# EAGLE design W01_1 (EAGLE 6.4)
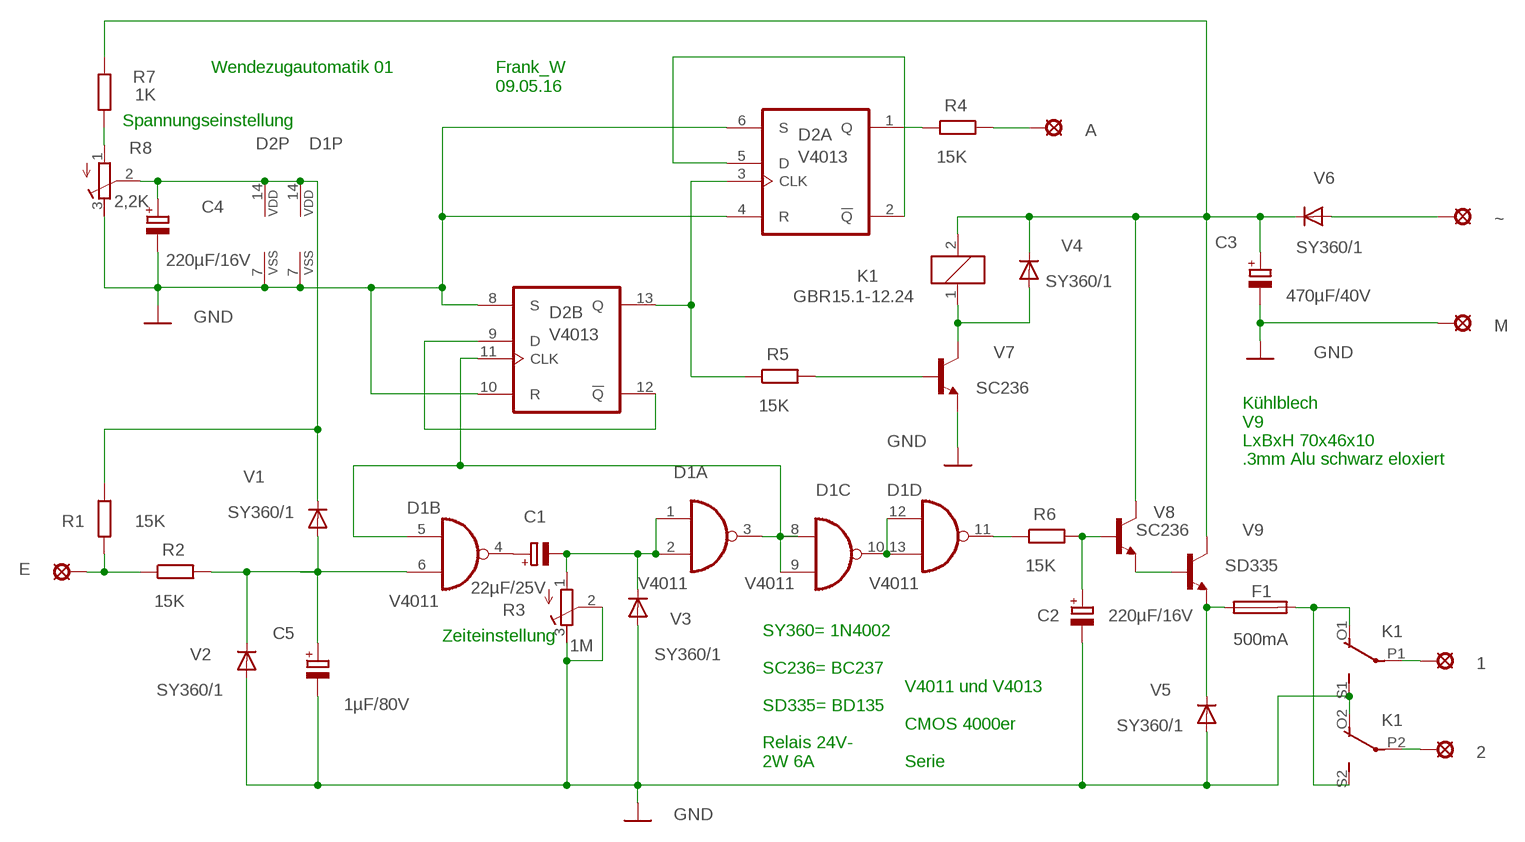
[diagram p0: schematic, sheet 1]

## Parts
1  LSP10  [LSP10]
2  LSP10  [LSP10]
A  LSP10  [LSP10]
C1  22µF/25V  CPOL-EUE5-5  [E5-5]
C2  220µF/16V  CPOL-EUE22-9AXIAL  [E22-9]
C3  470µF/40V  CPOL-EUE22-9AXIAL  [E22-9]
C4  220µF/16V  CPOL-EUE22-9AXIAL  [E22-9]
C5  1µF/80V  CPOL-EUE5-5  [E5-5]
D1  V4011  4011N  [DIL14]
D2  V4013  4013N  [DIL14]
E  LSP10  [LSP10]
F1  500mA  GSH15  [GSH15]
K1  GBR15.1-12.24  4052  [F4052]
M  LSP10  [LSP10]
R1  15K  R-EU_0207/12  [0207/12]
R2  15K  R-EU_0207/12  [0207/12]
R3  1M  R-TRIMM3296P  [RTRIM3296P]
R4  15K  R-EU_0207/12  [0207/12]
R5  15K  R-EU_0207/12  [0207/12]
R6  15K  R-EU_0207/12  [0207/12]
R7  1K  R-EU_0207/12  [0207/12]
R8  2,2K  R-TRIMM3296P  [RTRIM3296P]
V1  SY360/1  1N4004  [DO41-10]
V2  SY360/1  1N4004  [DO41-10]
V3  SY360/1  1N4004  [DO41-10]
V4  SY360/1  1N4004  [DO41-10]
V5  SY360/1  1N4004  [DO41-10]
V6  SY360/1  1N4004  [DO41-10]
V7  SC236  BC237  [TO92]
V8  SC236  BC237  [TO92]
V9  SD335  BD139  [TO126]
~  LSP10  [LSP10]

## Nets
GND: C2.- C3.- C4.- C5.- D1.7(P:VSS) D2.4(A:R) D2.6(A:S) D2.7(P:VSS) D2.8(B:S) D2.10(B:R) K1.O2(3:O) K1.S1(2:S) M.MP R3.2(S) R3.3(E) R8.3(E) V2.A V3.A V5.A V7.1(E)
N$1: E.MP R1.2 R2.1
N$2: C5.+ D1.6(B:I1) R2.2 V1.A V2.C
N$4: D2.9(B:D) D2.12(B:!Q)
N$6: D1.11(D:O) R6.1
N$7: C2.+ R6.2 V8.2(B)
N$8: R7.2 R8.1(A)
N$9: V6.A ~.MP
N$10: D1.10(C:O) D1.12(D:I0) D1.13(D:I1)
N$11: V8.1(E) V9.3(B)
N$12: F1.1 V5.C V9.1(E)
N$13: 1.MP K1.P1(2:P)
N$14: 2.MP K1.P2(3:P)
N$15: C1.- D1.1(A:I0) D1.2(A:I1) R3.1(A) V3.C
N$16: F1.2 K1.O1(2:O) K1.S2(3:S)
N$17: D1.3(A:O) D1.5(B:I0) D1.8(C:I0) D1.9(C:I1) D2.11(B:CLK)
N$18: D2.3(A:CLK) D2.13(B:Q) R5.1
N$19: C4.+ D1.14(P:VDD) D2.14(P:VDD) R1.1 R8.2(S) V1.C
N$20: R5.2 V7.2(B)
N$21: K1.1 V4.A V7.3(C)
N$22: D2.2(A:!Q) D2.5(A:D)
N$23: C3.+ K1.2 R7.1 V4.C V6.C V8.3(C) V9.2(C)
N$24: D2.1(A:Q) R4.1
N$26: A.MP R4.2
N$27: C1.+ D1.4(B:O)

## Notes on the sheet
- Wendezugautomatik 01
- Frank_W
  09.05.16
- Spannungseinstellung
- Kühlblech
  V9
  LxBxH 70x46x10
  .3mm Alu schwarz eloxiert
- Zeiteinstellung
- SY360= 1N4002
  
  SC236= BC237
  
  SD335= BD135
  
  Relais 24V-
  2W 6A
- V4011 und V4013
  
  CMOS 4000er
  
  Serie

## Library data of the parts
1 2 A E M ~ = solpad:LSP10: SOLDER PAD
C1-C5 = rcl:CPOL-EU: POLARIZED CAPACITOR, European symbol
D1 = 40xx:4011: Quad 2-input NAND
D2 = 40xx:4013: Dual D FLIP FLOP, set/reset
F1 = fuse:GSH15: FUSE HOLDER; MPN: 64900001039; OC_FARNELL: 1271673; OC_NEWARK: 02P0318
K1 = relay:4052: RELAY 2 x switch, Finder; OC_FARNELL: unknown; OC_NEWARK: unknown
R1 R2 R4-R7 = rcl:R-EU_: RESISTOR, European symbol
R3 R8 = rcl:R-TRIMM: Trimm resistor
V1-V6 = diode:1N4004: DIODE
V7 V8 = transistor-neu-to92:BC237: NPN TRANSISTOR
V9 = transistor:BD139: NPN TRANSISTOR

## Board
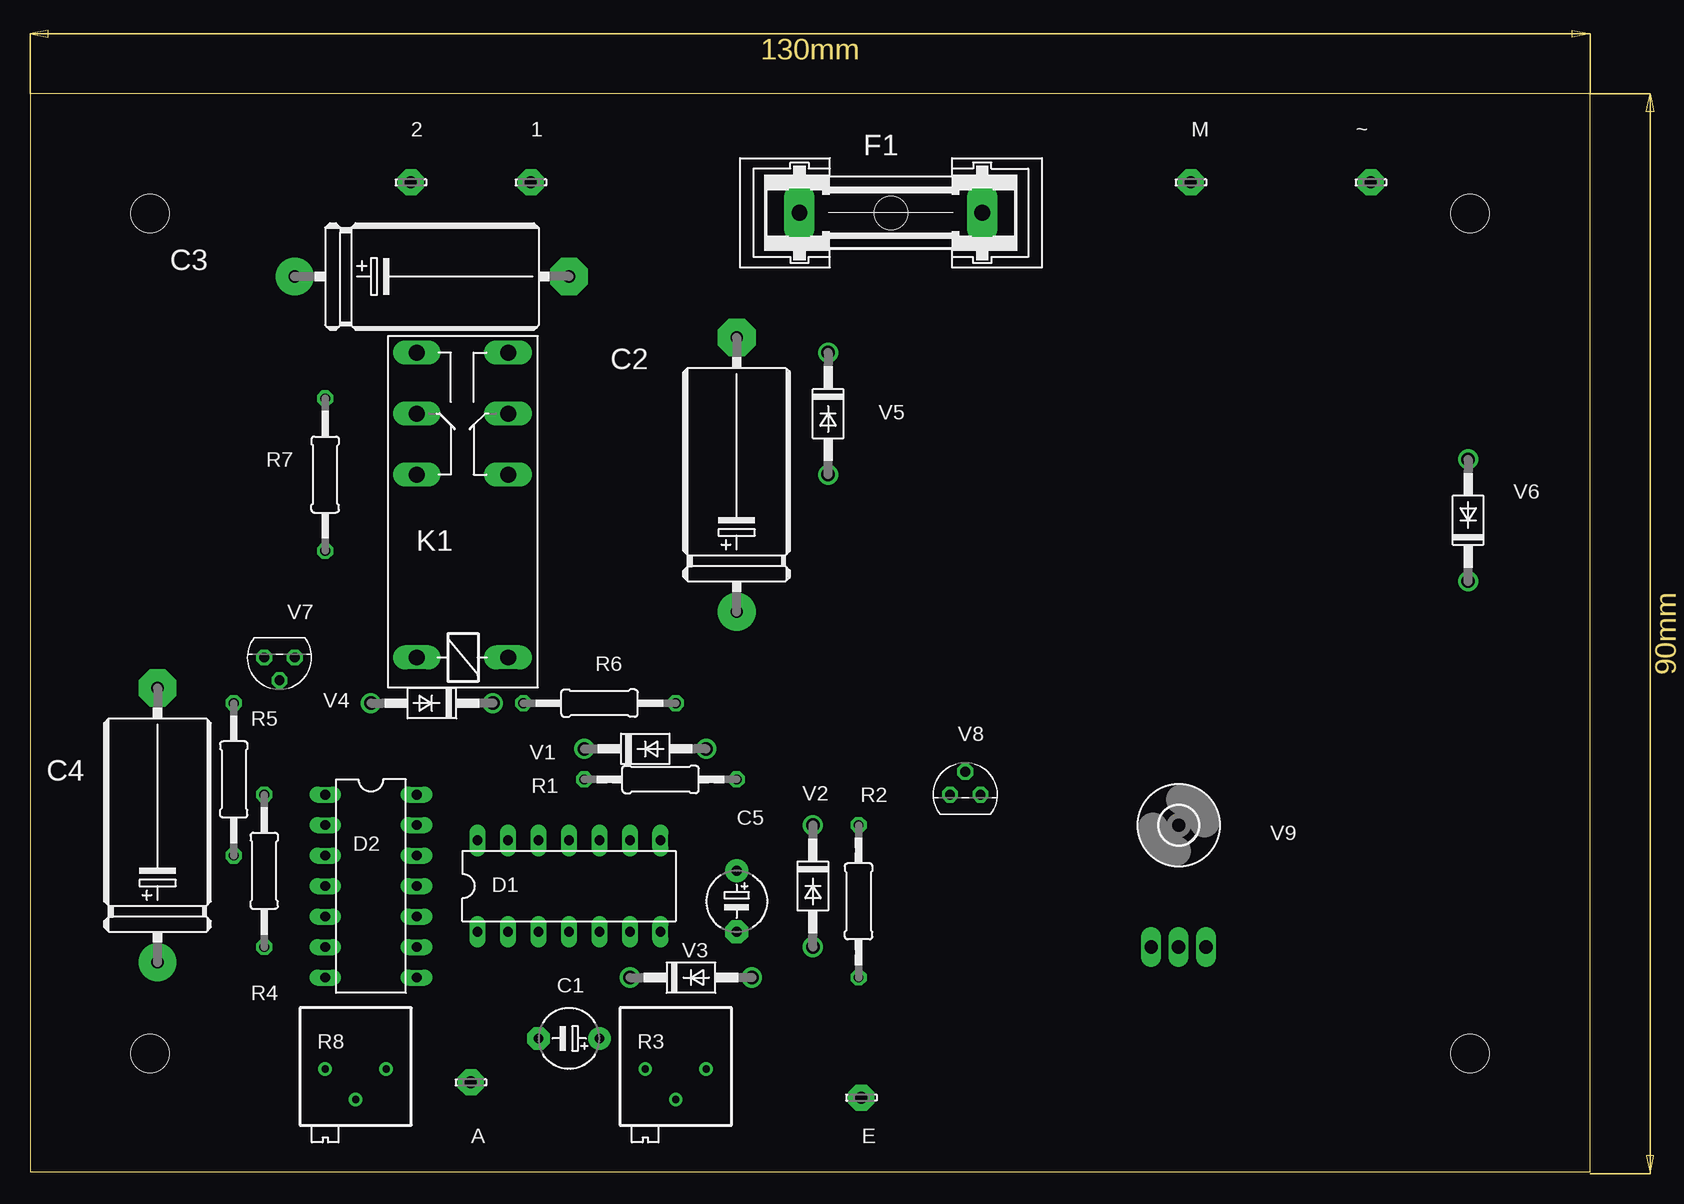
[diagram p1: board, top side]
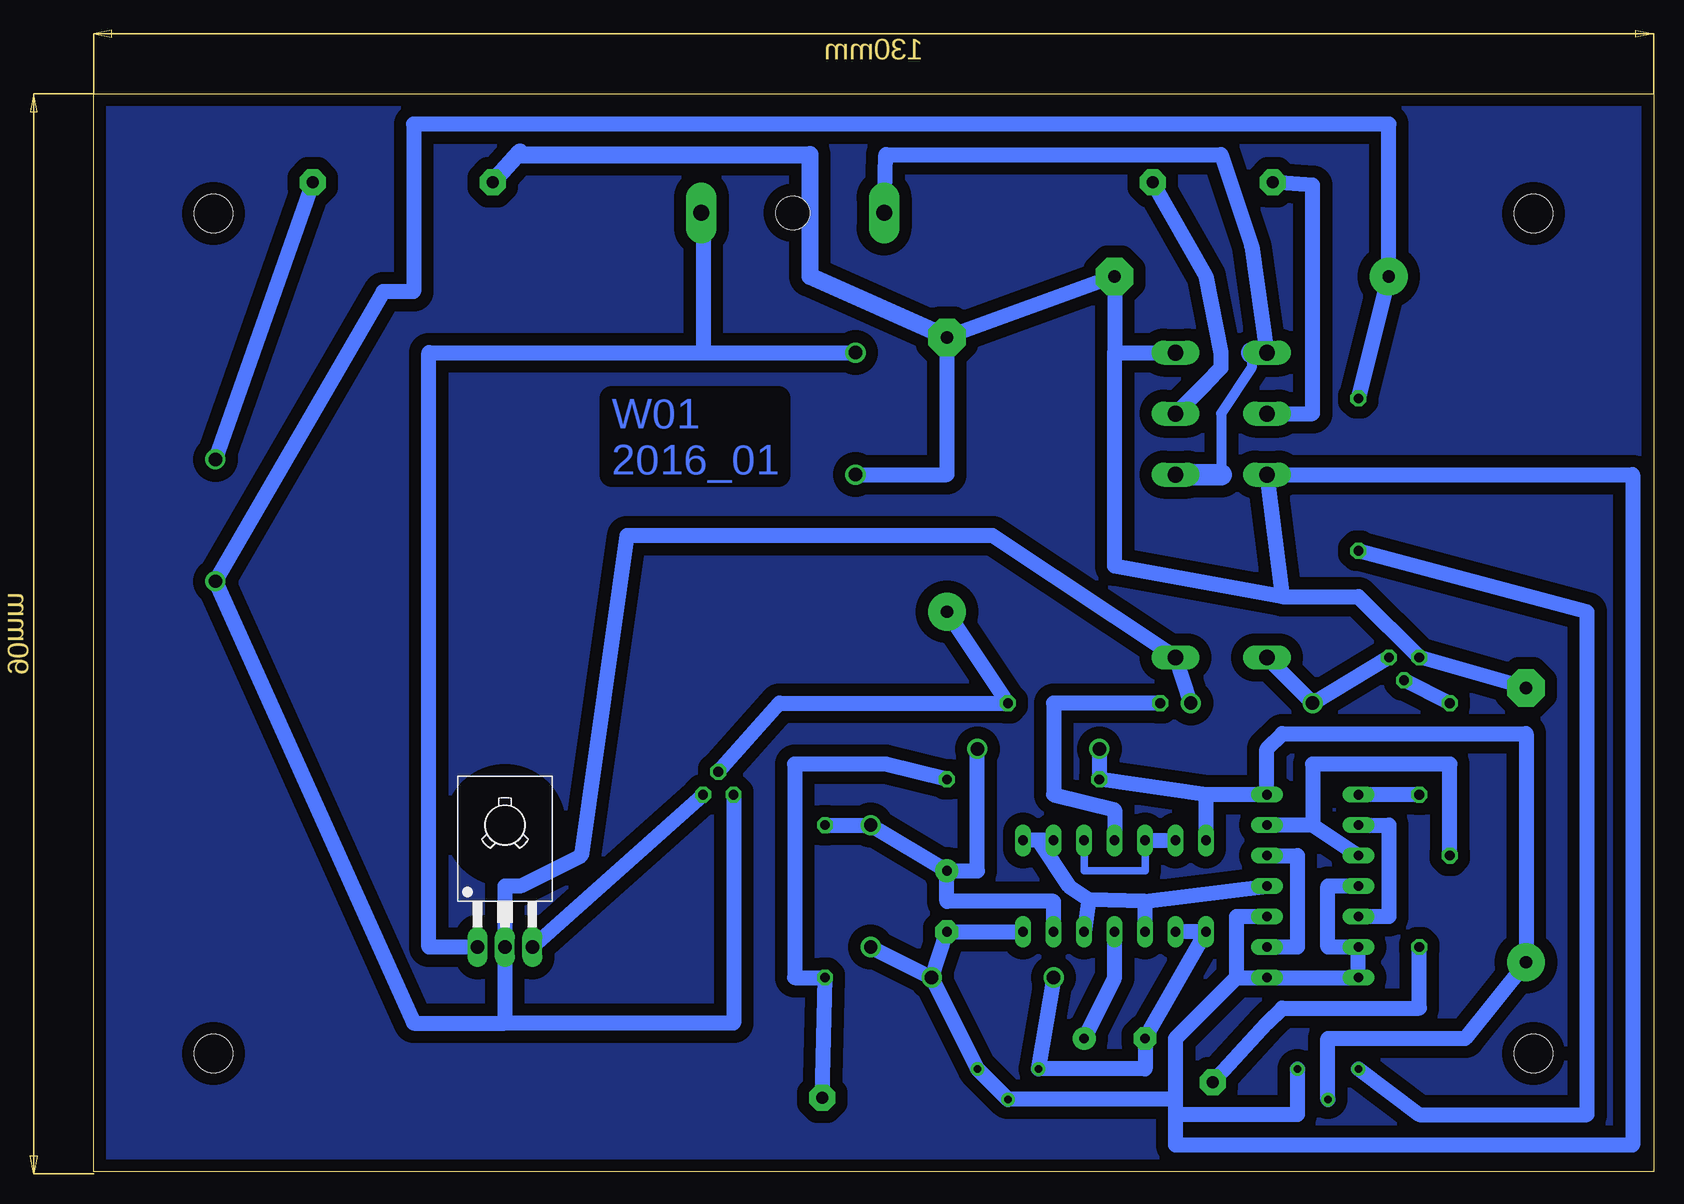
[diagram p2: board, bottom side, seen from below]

Size 135.3 x 95.3 mm. Coordinates in mm from the lower left corner, seen from the top.
Outline: 0,90 0,0.16 130,0.16 130,90 0,90
Copper layers (1*16): Top 0.035mm / dielectric 1.5mm / Bottom 0.035mm
Design rules "default *": minimum track width 20mil, minimum drill 24mil, track to track 8mil, track to pad 8mil, pad to pad 8mil, via to via 8mil, smd to smd 8mil, copper to edge 40mil, drill to drill 8mil, minimum pad ring 10mil, minimum via ring 8mil, stop-mask expansion 4mil, vias tented up to drill 0mil, thermal gap 20mil
Holes 3.2 mm at 120,10 10,10 10,80 120,80

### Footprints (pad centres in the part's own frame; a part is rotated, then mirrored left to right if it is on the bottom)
LSP10 = drill 1.016 pad 2.159 octagon: MP 0,0
E5-5 = drill 0.813 pad 1.905: + -2.54,0 | drill 0.813 pad 1.905 octagon: - 2.54,0
E22-9 = drill 1.016 pad 3.15: + -11.43,0 | drill 1.016 pad 3.15 octagon: - 11.43,0
DIL14 = drill 0.813 long: 1 -7.62,-3.81; 2 -5.08,-3.81; 3 -2.54,-3.81; 4 0,-3.81; 5 2.54,-3.81; 6 5.08,-3.81; 7 7.62,-3.81; 8 7.62,3.81; 9 5.08,3.81; 10 2.54,3.81; 11 0,3.81; 12 -2.54,3.81; 13 -5.08,3.81; 14 -7.62,3.81
GSH15 = drill 1.321 pad 2.54 long: 1 -7.62,0; 2 7.62,0 | hole 2.794: 0,0
F4052 = drill 1.321 long: 1 -3.81,3.81; 2 -3.81,-3.81; O1 11.43,-3.81; O2 11.43,3.81; P1 16.51,-3.81; P2 16.51,3.81; S1 21.59,-3.81; S2 21.59,3.81
0207/12 = drill 0.813 octagon: 1 -6.35,0; 2 6.35,0
RTRIM3296P = drill 0.61: 1 0,-2.54; 2 2.54,0; 3 0,2.54
3,2 = hole 3.2: 0,0
DO41-10 = drill 1.118: A 5.08,0; C -5.08,0
TO92 = drill 0.813 octagon: 1 1.27,0; 2 0,1.905; 3 -1.27,0
TO126 = drill 1.118 long: 1 -2.286,-5.08; 2 0,-5.08; 3 2.286,-5.08 | hole 3.302: 0,5.08

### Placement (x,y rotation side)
1  41.74,82.6 0 top
2  31.74,82.6 0 top
A  36.74,7.6 0 top
C1  44.92,11.26 180 top
C2  58.89,58.25 90 top
C3  33.49,74.76 0 top
C4  10.63,29.04 90 top
C5  58.89,22.69 270 top
D1  44.92,23.96 0 top
D2  28.41,23.96 270 top
E  69.28,6.33 0 top
F1  71.74,80.06 180 top
K1  36.03,46.82 90 top
M  96.74,82.6 0 top
R1  52.54,32.85 0 top
R2  69.05,22.69 90 top
R3  53.81,8.72 270 top
R4  19.52,25.23 270 top
R5  16.98,32.85 90 top
R6  47.46,39.2 0 top
R7  24.6,58.25 270 top
R8  27.14,8.72 270 top
U$1  [3,2]  95.72,29.04 0 top
V1  51.27,35.39 0 top
V2  65.24,23.96 270 top
V3  55.08,16.34 0 top
V4  33.49,39.2 180 top
V5  66.51,63.33 270 top
V6  119.85,54.44 90 top
V7  20.79,43.01 180 top
V8  77.94,31.58 0 top
V9  95.72,23.96 0 bottom
~  111.74,82.6 0 top

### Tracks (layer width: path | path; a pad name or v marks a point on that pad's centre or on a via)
GND
  Bottom 1.27: V3.A R3.3 R3.2 39.84,6.18 | V3.A V2.A | V3.A C5.- D1.7 | 44.92,68.41 C3.- C2.- 58.89,58.25 V5.A | 44.92,68.41 K1.S1 | D2.10 34.76,21.42 34.76,16.34 | 34.76,16.34 D2.8 D2.7 D2.6 27.14,18.88 27.14,23.96 D2.4 | R8.3 29.68,4.91 39.84,4.91 | 39.84,4.91 39.84,6.18 | 39.84,6.18 39.84,11.26 34.76,16.34 | 30.95,48.09 K1.O2 1.74,58.25 1.74,2.37 39.84,2.37 39.84,4.91 | 30.95,48.09 44.92,50.63 44.92,68.41 | 30.95,48.09 24.6,48.09 V7.1 C4.-
  Bottom 1.422: M.MP 94.45,85.14 94.45,84.92 70.32,84.92 70.32,74.76 C2.-
N$1
  Bottom 1.27: E.MP R2.1 71.59,16.34 71.59,34.12 63.97,34.12 R1.2
N$2
  Bottom 1.27: R2.2 V2.C C5.+ | C5.+ 56.35,25.23 V1.A | D1.6 50,22.69 58.89,22.69 C5.+
N$3
  pour Bottom (isolate 1.016): 0.47,90 130.01,90 130.01,-0.17 0.47,-0.17
N$4
  Bottom 1.27: D2.12 29.68,26.5 29.68,18.88 D2.9
N$6
  Bottom 1.27: R6.1 50,39.2 50,31.58 44.92,30.31 D1.11
N$7
  Bottom 1.27: C2.+ R6.2 72.86,39.2 V8.2
N$8
  Bottom 1.27: R8.1 19.52,4.91 5.55,4.91 5.55,46.82 R7.2
N$9
  Bottom 1.27: ~.MP V6.A
N$10
  Bottom 0.61: D1.10 47.46,25.23 42.38,25.23 D1.12
  Bottom 1.27: D1.12 D1.13
N$11
  Bottom 1.27: V9.3 V8.1
N$12
  Bottom 1.016: F1.1 79.21,81.33
  Bottom 1.27: V9.1 102.07,18.88 102.07,68.41 79.21,68.41 | 79.21,68.41 V5.C | 79.21,81.33 79.21,68.41
N$13
  Bottom 1.27: K1.P1 37.3,65.87 36.03,67.14 36.03,68.41 37.3,74.76 1.MP
N$14
  Bottom 1.27: K1.P2 28.41,63.33 28.41,82.38 2.MP
N$15
  Bottom 1.27: V3.C R3.1 42.38,8.72 C1.- D1.1 D1.2
N$16
  Bottom 0.813: 33.49,68.41 33.49,67.14 36.03,63.33 36.03,58.25
  Bottom 1.27: F1.2 63.97,84.92 36.03,84.92 33.49,77.3 K1.S2
  Bottom 1.778: K1.S2 33.49,68.41 | 36.03,58.25 K1.O1
N$17
  Bottom 1.27: D1.9 51.27,27.77 | 51.27,27.77 D1.8 | 51.27,27.77 48.73,23.96 47.08,22.82 | 47.08,22.82 D1.5 | D1.3 42.38,22.69 | 42.38,22.69 47.08,22.82 | 42.38,22.69 D2.11
N$18
  Bottom 1.27: R5.1 16.98,34.12 28.41,34.12 28.41,29.04 | 28.41,29.04 D2.13 | 28.41,29.04 D2.3
N$19
  Bottom 1.27: V1.C R1.1 37.3,31.58 | R8.2 27.14,11.26 15.71,11.26 C4.+ 10.63,36.66 30.95,36.66 32.22,35.39 D2.14 37.3,31.58 | D1.14 37.3,31.58
N$20
  Bottom 1.27: R5.2 V7.2
N$21
  Bottom 1.27: V7.3 V4.A K1.1
N$22
  Bottom 1.27: D2.2 22.06,29.04 22.06,21.42 D2.5
N$23
  Bottom 1.27: 95.72,12.53 103.34,12.53 V6.C 105.88,73.49 103.34,73.49 103.34,87.46 22.06,87.46 C3.+ R7.1 | 95.72,12.53 V9.2 95.72,23.96 94.45,23.96 89.37,26.5 85.56,53.17 55.08,53.17 K1.2 V4.C | V8.3 76.67,12.53 95.72,12.53
N$24
  Bottom 1.27: R4.1 D2.1
N$26
  Bottom 1.27: A.MP 32.22,12.53 30.95,13.8 19.52,13.8 R4.2
N$27
  Bottom 1.27: C1.+ 44.92,16.34 D1.4

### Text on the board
Bottom: W01 / 2016_01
